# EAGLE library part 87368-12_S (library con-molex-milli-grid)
RECEPTACAL
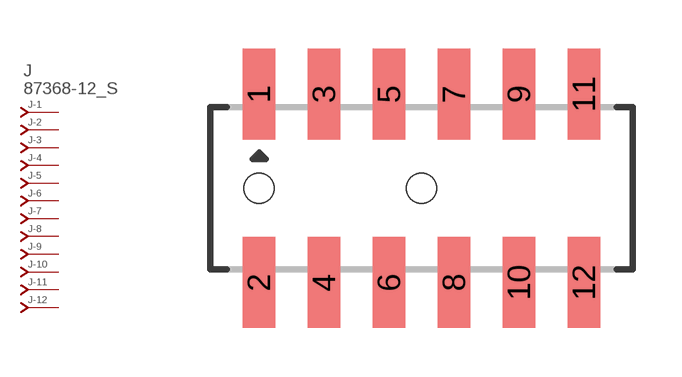
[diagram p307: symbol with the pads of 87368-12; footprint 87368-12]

Designator prefix J; gates -1=J-NV -2=J-N -3=J-N -4=J-N -5=J-N -6=J-N -7=J-N -8=J-N -9=J-N -10=J-N -11=J-N -12=J-N

## 87368-12_S  [87368-12]
1  -1:J  pas
2  -2:J  pas
3  -3:J  pas
4  -4:J  pas
5  -5:J  pas
6  -6:J  pas
7  -7:J  pas
8  -8:J  pas
9  -9:J  pas
10  -10:J  pas
11  -11:J  pas
12  -12:J  pas

## Footprint 87368-12 (pad centres in mm)
RECEPTACAL SMD Dual Row, Side Entry
smd 1 x 2.8: 1 -5,2.9; 2 -5,-2.9; 3 -3,2.9; 4 -3,-2.9; 5 -1,2.9; 6 -1,-2.9; 7 1,2.9; 8 1,-2.9; 9 3,2.9; 10 3,-2.9; 11 5,2.9; 12 5,-2.9
hole 0.914 at -5,0
hole 0.914 at 0,0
